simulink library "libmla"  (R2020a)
settings: Solver=ode45  StartTime=0.0  StopTime=10.0  RelTol=1e-3  EnableMultiTasking=on
libraries: simulink x3, xpcnilib x2

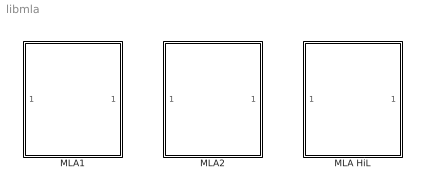
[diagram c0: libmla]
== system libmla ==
  MLA HiL : Subsystem
  MLA1 : Subsystem  mask(MLA - simple){g=9.81, m=0.125, d_l=0.5, a=40691, b=0.0687, N=4.282}
      mask prompts: g "Erdbeschleunigung"; m "Masse des Magneten"; d_l "Laminarer Reibungsbeiwert"; a "Kraftparameter a"; b "Kraftparameter b"; N "Kraftexponent"
      mask help: einfaches Modell des MLA 730
  MLA2 : Subsystem  mask(MLA){g=9.81, m=0.125, Fr_g=0.14, Fr_h=0.1, d_l=0.14, d_t=0.09, a=40691, b=0.0687, N=4.282}
      mask prompts: g "Erdbeschleunigung"; m "Masse des Magneten"; Fr_g "Gleitreibungskraft"; Fr_h "Haftreibungskraft"; d_l "Laminarer Reibungsbeiwert"; d_t "Turbulenter Reibungsbeiwert"; a "Kraftparameter a"; b "Kraftparameter b"; N "Kraftexponent"
      mask help: Modell des MLA 730 mit komplexem Reibungsmodell

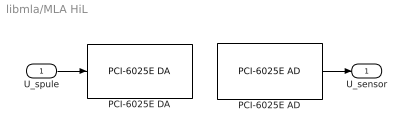
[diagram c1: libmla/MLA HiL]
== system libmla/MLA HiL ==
  U_spule : Inport
  PCI-6025E AD : xpcnilib/A//D/E Series/PCI-6025E AD  channel=[1]  range=[-10]  coupling=[0]  sampletime=0.0001  slot=-1
  PCI-6025E DA : xpcnilib/D//A/E Series/PCI-6025E DA  channel=[1]  reset=[1]  initValue=[0]  sampletime=0.0001  slot=-1
  U_sensor : Outport
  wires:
  PCI-6025E AD/1 -> U_sensor/1
  U_spule/1 -> PCI-6025E DA/1

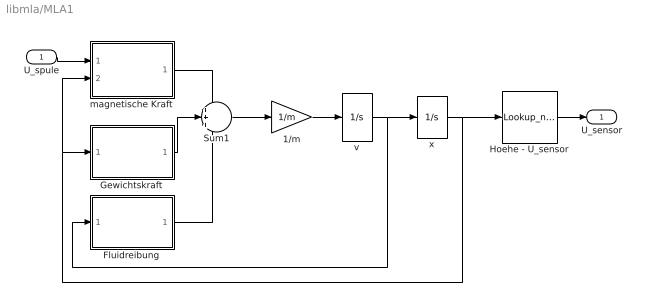
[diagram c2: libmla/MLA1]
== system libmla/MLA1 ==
  U_spule : Inport
  1/m : Gain  Gain=1/m
  Fluidreibung : Subsystem  mask{d_l=d_l}
      mask prompts: d_l "laminarer Reibungskoeffizient"
  Gewichtskraft : Subsystem  mask{m=m, g=g}
      mask prompts: m "Masse"; g "Erdbeschleunigung"
  Hoehe - U_sensor : Lookup_n-D  NumberOfTableDimensions=1  BreakpointsForDimension1=MLA_Sensor1(end:-1:1,2)  Table=MLA_Sensor1(end:-1:1,1)  RndMeth=Simplest
  Sum1 : Sum  Inputs=+++
  magnetische Kraft : Subsystem  mask{a=a, b=b, N=N}
      mask prompts: a "Kraftparameter a"; b "Kraftparameter b"; N "Exponent N"
  v : Integrator
  x : Integrator  LimitOutput=on  LowerSaturationLimit=0
  U_sensor : Outport
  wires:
  Fluidreibung/1(Fv) -> Sum1/3
  1/m/1 -> v/1
  v/1 -> x/1, Fluidreibung/1(v)
  Hoehe - U_sensor/1 -> U_sensor/1
  x/1 -> Hoehe - U_sensor/1, magnetische Kraft/2(x), Gewichtskraft/1(x)
  U_spule/1 -> magnetische Kraft/1(U_sp)
  Sum1/1 -> 1/m/1
  magnetische Kraft/1(F_M) -> Sum1/1
  Gewichtskraft/1(F_g) -> Sum1/2

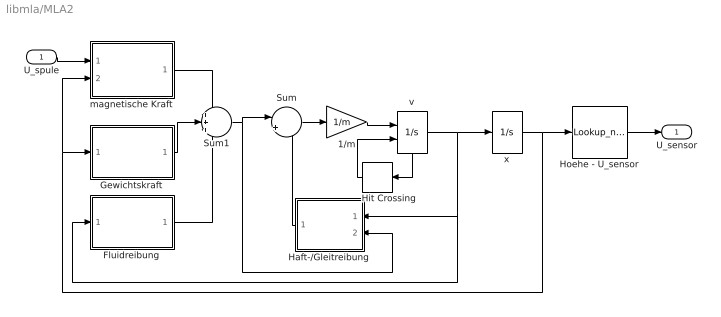
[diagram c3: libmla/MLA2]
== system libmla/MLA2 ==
  U_spule : Inport
  1/m : Gain  Gain=1/m
  Fluidreibung : Subsystem  mask{d_l=d_l, d_t=d_t}
      mask prompts: d_l "laminarer Reibungskoeffizient"; d_t "turbulenter Reibungskoeffizient"
  Gewichtskraft : Subsystem  mask{m=m, g=g}
      mask prompts: m "Masse"; g "Erdbeschleunigung"
  Haft-/Gleitreibung : Subsystem  mask(Reibungskraft){mug=Fr_g, muh=Fr_h, FN=1}
      mask prompts: mug "Gleitreibungskoeffizient"; muh "Haftreibungskoeffizient"; FN "Normalkraft"
      mask help: Berechnet die Reibungskraft fuer Haft- und Gleitreibung. Eingaenge: Geschwindigkeit, aeussere Kraft.
  Hit Crossing : HitCross
  Hoehe - U_sensor : Lookup_n-D  NumberOfTableDimensions=1  BreakpointsForDimension1=MLA_Sensor1(end:-1:1,2)  Table=MLA_Sensor1(end:-1:1,1)  RndMeth=Simplest
  Sum : Sum  Inputs=|++
  Sum1 : Sum  Inputs=+++
  magnetische Kraft : Subsystem  mask{a=a, b=b, N=N}
      mask prompts: a "Kraftparameter a"; b "Kraftparameter b"; N "Exponent N"
  v : Integrator  ExternalReset=rising  ShowStatePort=on
  x : Integrator  LimitOutput=on  LowerSaturationLimit=0
  U_sensor : Outport
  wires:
  Hit Crossing/1 -> v/2
  Gewichtskraft/1(F_g) -> Sum1/2
  magnetische Kraft/1(F_M) -> Sum1/1
  Sum1/1 -> Haft-/Gleitreibung/2(F_ext), Sum/1
  Sum/1 -> 1/m/1
  U_spule/1 -> magnetische Kraft/1(U_sp)
  x/1 -> Gewichtskraft/1(x), magnetische Kraft/2(x), Hoehe - U_sensor/1
  Hoehe - U_sensor/1 -> U_sensor/1
  v/1 -> x/1, Haft-/Gleitreibung/1(v), Fluidreibung/1(v)
  1/m/1 -> v/1
  Fluidreibung/1(Fv) -> Sum1/3
  Haft-/Gleitreibung/1(F_R) -> Sum/2
  v/State -> Hit Crossing/1

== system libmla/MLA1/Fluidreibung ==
  v : Inport
  Unary Minus : UnaryMinus
  laminar : Gain  Gain=d_l
  Fv : Outport
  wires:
  v/1 -> laminar/1
  laminar/1 -> Unary Minus/1
  Unary Minus/1 -> Fv/1

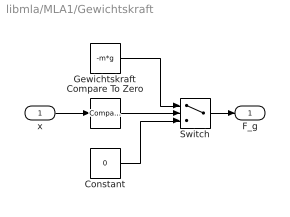
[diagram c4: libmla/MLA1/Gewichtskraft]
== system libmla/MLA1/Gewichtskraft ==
  x : Inport
  Compare To Zero : simulink/Logic and Bit Operations/Compare To Zero  SystemSampleTime=-1  relop=>  LogicOutDataTypeMode=boolean
  Constant : Constant  Value=0
  Gewichtskraft : Constant  Value=-m*g
  Switch : Switch  Criteria=u2 > Threshold  Threshold=0.5
  F_g : Outport
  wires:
  Compare To Zero/1 -> Switch/2
  Gewichtskraft/1 -> Switch/1
  Constant/1 -> Switch/3
  x/1 -> Compare To Zero/1
  Switch/1 -> F_g/1

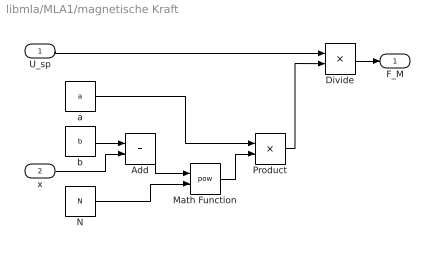
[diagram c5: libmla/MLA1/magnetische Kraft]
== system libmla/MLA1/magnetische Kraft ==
  U_sp : Inport
  x : Inport  Port=2
  Add : Sum
  Divide : Product  Inputs=*/
  Math Function : Math  Operator=pow  SignedPower=on
  N : Constant  Value=N
  Product : Product  RndMeth=Zero
  a : Constant  Value=a
  b : Constant  Value=b
  F_M : Outport
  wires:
  N/1 -> Math Function/2
  Add/1 -> Math Function/1
  x/1 -> Add/2
  b/1 -> Add/1
  Math Function/1 -> Product/2
  a/1 -> Product/1
  Product/1 -> Divide/2
  U_sp/1 -> Divide/1
  Divide/1 -> F_M/1

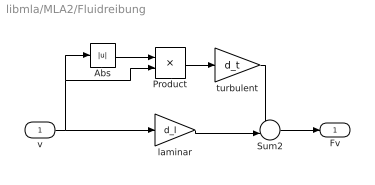
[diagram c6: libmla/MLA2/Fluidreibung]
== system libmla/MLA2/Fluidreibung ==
  v : Inport
  Abs : Abs
  Product : Product  RndMeth=Zero
  Sum2 : Sum  Inputs=--|
  laminar : Gain  Gain=d_l
  turbulent : Gain  Gain=d_t
  Fv : Outport
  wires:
  laminar/1 -> Sum2/2
  turbulent/1 -> Sum2/1
  Product/1 -> turbulent/1
  Abs/1 -> Product/1
  v/1 -> Product/2, Abs/1, laminar/1
  Sum2/1 -> Fv/1

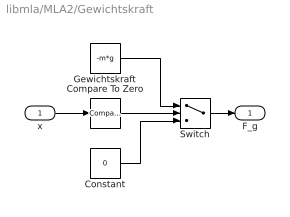
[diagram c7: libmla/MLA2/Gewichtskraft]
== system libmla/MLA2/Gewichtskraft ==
  x : Inport
  Compare To Zero : simulink/Logic and Bit Operations/Compare To Zero  SystemSampleTime=-1  relop=>  LogicOutDataTypeMode=boolean
  Constant : Constant  Value=0
  Gewichtskraft : Constant  Value=-m*g
  Switch : Switch  Criteria=u2 > Threshold  Threshold=0.5
  F_g : Outport
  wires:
  Switch/1 -> F_g/1
  x/1 -> Compare To Zero/1
  Constant/1 -> Switch/3
  Gewichtskraft/1 -> Switch/1
  Compare To Zero/1 -> Switch/2

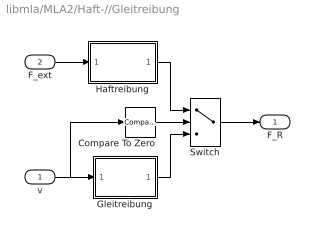
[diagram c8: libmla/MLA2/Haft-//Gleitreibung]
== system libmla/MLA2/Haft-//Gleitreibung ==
  v : Inport
  F_ext : Inport  Port=2
  Compare To Zero : simulink/Logic and Bit Operations/Compare To Zero  SystemSampleTime=-1  relop===  LogicOutDataTypeMode=uint8
  Gleitreibung : Subsystem
  Haftreibung : Subsystem
  Switch : Switch  Criteria=u2 ~= 0  Threshold=0.5
  F_R : Outport
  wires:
  Switch/1 -> F_R/1
  F_ext/1 -> Haftreibung/1(F_ext)
  v/1 -> Compare To Zero/1, Gleitreibung/1(v)
  Haftreibung/1(F_h) -> Switch/1
  Gleitreibung/1(F_g) -> Switch/3
  Compare To Zero/1 -> Switch/2

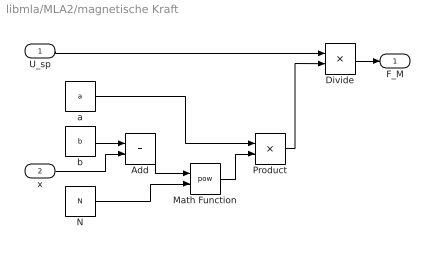
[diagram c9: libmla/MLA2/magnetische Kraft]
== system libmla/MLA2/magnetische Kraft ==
  U_sp : Inport
  x : Inport  Port=2
  Add : Sum
  Divide : Product  Inputs=*/
  Math Function : Math  Operator=pow  SignedPower=on
  N : Constant  Value=N
  Product : Product  RndMeth=Zero
  a : Constant  Value=a
  b : Constant  Value=b
  F_M : Outport
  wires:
  Divide/1 -> F_M/1
  U_sp/1 -> Divide/1
  Product/1 -> Divide/2
  a/1 -> Product/1
  Math Function/1 -> Product/2
  b/1 -> Add/1
  x/1 -> Add/2
  Add/1 -> Math Function/1
  N/1 -> Math Function/2

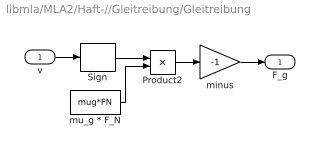
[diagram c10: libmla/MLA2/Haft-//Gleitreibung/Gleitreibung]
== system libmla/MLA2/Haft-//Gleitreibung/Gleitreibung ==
  v : Inport
  Product2 : Product  InputSameDT=on  SaturateOnIntegerOverflow=on
  Sign : Signum
  minus : Gain  Gain=-1  SaturateOnIntegerOverflow=on
  mu_g * F_N : Constant  Value=mug*FN
  F_g : Outport
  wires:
  mu_g * F_N/1 -> Product2/2
  Sign/1 -> Product2/1
  v/1 -> Sign/1
  Product2/1 -> minus/1
  minus/1 -> F_g/1

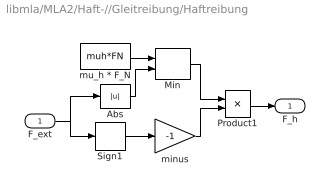
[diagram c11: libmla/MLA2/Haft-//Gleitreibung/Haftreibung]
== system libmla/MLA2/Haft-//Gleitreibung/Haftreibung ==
  F_ext : Inport
  Abs : Abs
  Min : MinMax  Inputs=2  InputSameDT=on  SaturateOnIntegerOverflow=on
  Product1 : Product  InputSameDT=on  SaturateOnIntegerOverflow=on
  Sign1 : Signum
  minus : Gain  Gain=-1  SaturateOnIntegerOverflow=on
  mu_h * F_N : Constant  Value=muh*FN
  F_h : Outport
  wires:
  Abs/1 -> Min/2
  mu_h * F_N/1 -> Min/1
  Min/1 -> Product1/1
  F_ext/1 -> Abs/1, Sign1/1
  Product1/1 -> F_h/1
  Sign1/1 -> minus/1
  minus/1 -> Product1/2
